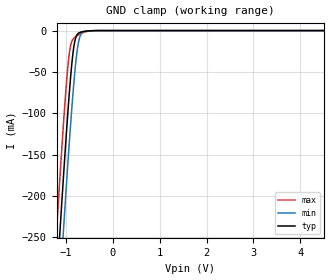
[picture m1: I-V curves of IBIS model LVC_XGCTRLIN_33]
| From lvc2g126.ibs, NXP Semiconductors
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| Remark: If your software does not support the Model Selector
|   Please comment out the lines of the Model Selector, which
|   contain the name of the Model, except the one you want to use.
|   Model LVC_XGCTRLIN_33
[Model]   LVC_XGCTRLIN_33
Model_type   Input
Vinl =   0.8V
Vinh =   2.0V
C_comp   2.9214pF   2.1165pF   3.8736pF
|Ambient temperature:   25   85   -40
[Temperature Range]   50   105   -10
[Voltage Range]   3.3V   3.0V   3.6V
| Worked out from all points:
|   GND clamp passes 1 mA (typ) near -0.61 V on its own axis
|Process Range   nominal   slow   fast
[GND_clamp]
| voltage   I(typ)   I(min)   I(max)
-5.5V     -4.538A    -4.596A    -4.481A
-1.208V   -316.9mA   -382.8mA   -250.3mA
-1.142V   -256.6mA   -322.3mA   -190.4mA
-1.12V    -236.8mA   -302.4mA   -170.9mA
-1.054V   -178.5mA   -243.3mA   -114.3mA
-988mV    -122.7mA   -185.9mA   -63.06mA
-922mV    -71.73mA   -131.2mA   -25.25mA
-812mV    -13.3mA    -51.49mA   -8.276mA
-746mV    -3.802mA   -18.87mA   -5.651mA
-702mV    -2.246mA   -7.433mA   -4.219mA
-400mV    -94.75uA   -95.65uA   -83.86uA
5.5V      0A         0A         0A
